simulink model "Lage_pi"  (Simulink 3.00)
settings: Solver=ode5  SolverMode=SingleTasking  StartTime=0.0  StopTime=1.75  RelTol=1e-3  AbsTol=1e-6
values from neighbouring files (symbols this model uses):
  bm = 4    [PI_Par.m]    (also in Red_Par.m)
  K_St = 1/FD_Stern    (= 2.27848101266)    [PI_Par.m]    (also in Red_Par.m = 1/FD_Stern)
  KL = omd*sqrt((1-TR^2*omd^2)+4*dR^2*TR^2*omd^2)    [PI_Par.m]    (also in Red_Par.m)
  KP = (1/K_St)*(2*d*T_St-T)/T    (= 23.3767988889)    [PI_Par.m]
  KVor = 1    [PI_Par.m]    (also in Red_Par.m)
  qA = 0    [PI_Par.m]    (also in Red_Par.m)
  T_St = M_Stern/FD_Stern    (= 2.82860759494)    [PI_Par.m]    (also in Red_Par.m = M_Stern/FD_Stern)
  tb = vm/bm    (= 0.5)    [PI_Par.m]    (also in Red_Par.m)
  te = tv+tb    (= 1.2853981634)    [PI_Par.m]    (also in Red_Par.m)
  TN = T*(2*d-T/T_St)    (= 0.0693971006366)    [PI_Par.m]
  tv = se/vm    (= 0.785398163397)    [PI_Par.m]    (also in Red_Par.m)
  Vorz = 1    [PI_Par.m]    (also in Red_Par.m)
  z0 = (1/KM)*(rh)    (= 1.25)    [PI_Par.m]    (also in Red_Par.m = (1/KM)*(rh))

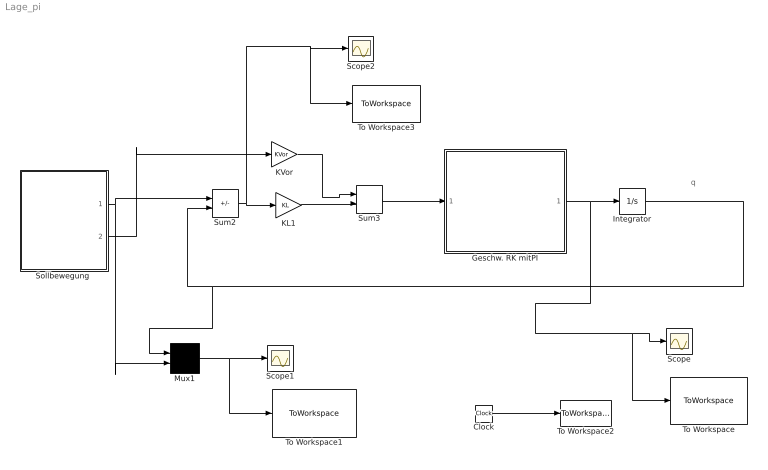
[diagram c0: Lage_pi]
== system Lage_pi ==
  note: q
  Clock : Clock
  Geschw. RK mitPI : Subsystem
  Integrator : Integrator  ExternalReset=none  InitialConditionSource=internal  InitialCondition=0  LimitOutput=off  UpperSaturationLimit=inf  LowerSaturationLimit=-inf  ShowSaturationPort=off  ShowStatePort=off  AbsoluteTolerance=auto
  KL1 : Gain  Gain=KL  SaturateOnIntegerOverflow=on
  KVor : Gain  Gain=KVor  SaturateOnIntegerOverflow=on
  Mux1 : Mux  Inputs=2
  Scope : Scope
  Scope1 : Scope
  Scope2 : Scope
  "Sollbewegung " : Subsystem
  Sum2 : Sum  Inputs=+-  SaturateOnIntegerOverflow=on
  Sum3 : Sum  Inputs=++  SaturateOnIntegerOverflow=on
  To Workspace : ToWorkspace  VariableName=Geschw_PI_M_Max  SampleTime=0.001  SaveFormat=Matrix
  To Workspace1 : ToWorkspace  VariableName=Lage_PI_M_Max  SampleTime=0.001  SaveFormat=Matrix
  To Workspace2 : ToWorkspace  VariableName=Zeit_Lage  SampleTime=0.001  SaveFormat=Matrix
  To Workspace3 : ToWorkspace  VariableName=e_PI_M_Max  SampleTime=0.001  SaveFormat=Matrix
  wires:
  Clock/1 -> To Workspace2/1
  KL1/1 -> Sum3/2
  KVor/1 -> Sum3/1
  Mux1/1 -> To Workspace1/1, Scope1/1
  "Sollbewegung "/1(qS) -> Sum2/1, Mux1/2
  Integrator/1 -> Sum2/2, Mux1/1
  Geschw. RK mitPI/1(v) -> Integrator/1, Scope/1, To Workspace/1
  Sum2/1 -> KL1/1, Scope2/1, To Workspace3/1
  Sum3/1 -> Geschw. RK mitPI/1(qps)
  "Sollbewegung "/2(qpss) -> KVor/1

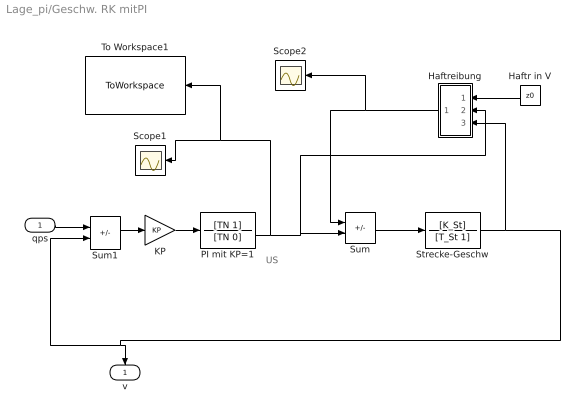
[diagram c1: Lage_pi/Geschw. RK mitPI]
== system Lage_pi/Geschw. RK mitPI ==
  note: US
  qps : Inport  Port=1  PortWidth=-1  SampleTime=-1  DataType=auto
  Haftr in V : Constant  Orientation=left  Value=z0
  Haftreibung : Subsystem  Orientation=left
  KP : Gain  Gain=KP  SaturateOnIntegerOverflow=on
  PI mit KP=1 : TransferFcn  Numerator=[TN 1]  Denominator=[TN 0]
  Scope1 : Scope
  Scope2 : Scope
  Strecke-Geschw : TransferFcn  Numerator=[K_St]  Denominator=[T_St 1]
  Sum : Sum  Inputs=-+  SaturateOnIntegerOverflow=on
  Sum1 : Sum  Inputs=+-  SaturateOnIntegerOverflow=on
  To Workspace1 : ToWorkspace  VariableName=Lage_PI_M_Max_US  SampleTime=0.001  SaveFormat=Matrix
  v : Outport  Orientation=down  Port=1
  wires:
  Sum1/1 -> KP/1
  KP/1 -> PI mit KP=1/1
  PI mit KP=1/1 -> Sum/2, Haftreibung/2(US), Scope1/1, To Workspace1/1
  Strecke-Geschw/1 -> Haftreibung/3(qp), Sum1/2, v/1
  Sum/1 -> Strecke-Geschw/1
  Haftr in V/1 -> Haftreibung/1(z0)
  Haftreibung/1(Out1) -> Sum/1, Scope2/1
  qps/1 -> Sum1/1

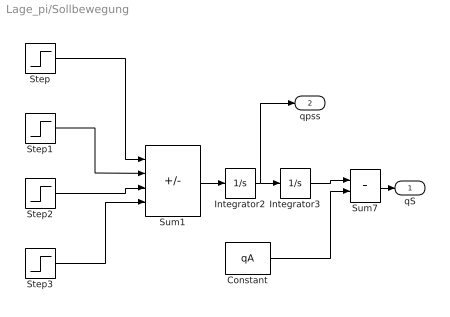
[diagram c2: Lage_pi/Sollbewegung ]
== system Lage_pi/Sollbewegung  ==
  Constant : Constant  Value=qA
  Integrator2 : Integrator  ExternalReset=none  InitialConditionSource=internal  InitialCondition=0  LimitOutput=off  UpperSaturationLimit=inf  LowerSaturationLimit=-inf  ShowSaturationPort=off  ShowStatePort=off  AbsoluteTolerance=auto
  Integrator3 : Integrator  ExternalReset=none  InitialConditionSource=internal  InitialCondition=0  LimitOutput=off  UpperSaturationLimit=inf  LowerSaturationLimit=-inf  ShowSaturationPort=off  ShowStatePort=off  AbsoluteTolerance=auto
  Step : Step  Time=0  Before=0  After=bm*Vorz  SampleTime=0.005
  Step1 : Step  Time=tb  Before=0  After=bm*Vorz  SampleTime=0.005
  Step2 : Step  Time=tv  Before=0  After=bm*Vorz  SampleTime=0.005
  Step3 : Step  Time=te  Before=0  After=bm*Vorz  SampleTime=0.005
  Sum1 : Sum  Inputs=+--+  SaturateOnIntegerOverflow=on
  Sum7 : Sum  Inputs=++  SaturateOnIntegerOverflow=on
  qS : Outport  Port=1  InitialOutput=0
  qpss : Outport  Port=2
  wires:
  Step/1 -> Sum1/1
  Step1/1 -> Sum1/2
  Step2/1 -> Sum1/3
  Step3/1 -> Sum1/4
  Sum1/1 -> Integrator2/1
  Integrator2/1 -> Integrator3/1, qpss/1
  Constant/1 -> Sum7/2
  Integrator3/1 -> Sum7/1
  Sum7/1 -> qS/1

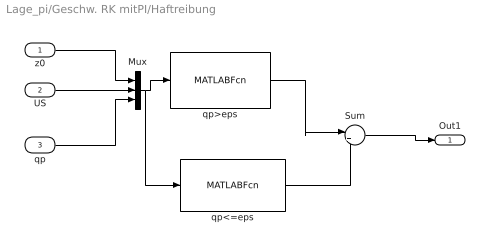
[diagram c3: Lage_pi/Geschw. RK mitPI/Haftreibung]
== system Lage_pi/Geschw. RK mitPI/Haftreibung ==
  z0 : Inport  Port=1  PortWidth=-1  SampleTime=-1  DataType=auto
  US : Inport  Port=2  PortWidth=-1  SampleTime=-1  DataType=auto
  qp : Inport  Port=3  PortWidth=-1  SampleTime=-1  DataType=auto
  Mux : Mux  Inputs=3
  Sum : Sum  Inputs=|++  SaturateOnIntegerOverflow=on
  qp<=eps : MATLABFcn  MATLABFcn=(abs(u(3)) < eps) *min(abs(u(2)),u(1))* sign(u(2))*sign(u(1))  OutputWidth=1  OutputSignalType=auto
  qp>eps : MATLABFcn  MATLABFcn=(abs(u(3)) > eps) * sign(u(3))*u(1)  OutputWidth=1  OutputSignalType=auto
  Out1 : Outport  Port=1  InitialOutput=0
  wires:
  z0/1 -> Mux/1
  US/1 -> Mux/2
  qp/1 -> Mux/3
  Mux/1 -> qp>eps/1, qp<=eps/1
  Sum/1 -> Out1/1
  qp>eps/1 -> Sum/1
  qp<=eps/1 -> Sum/2
